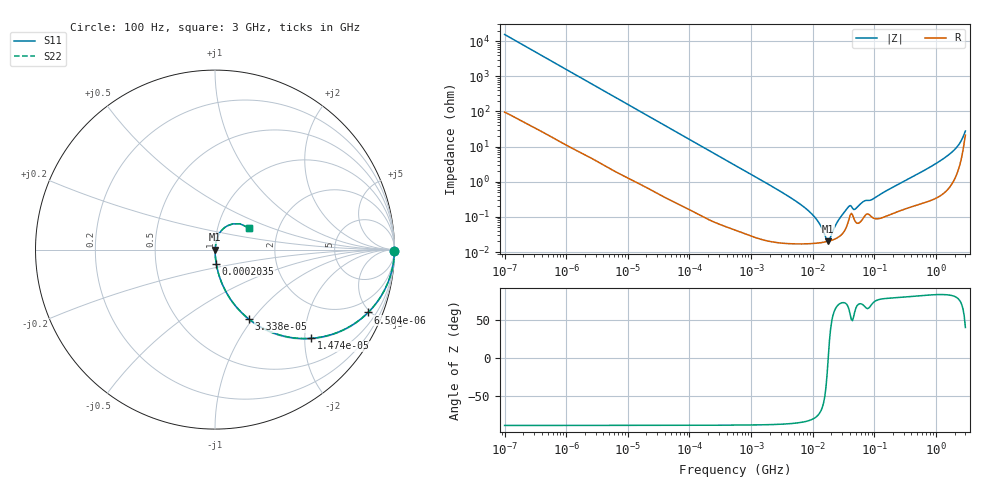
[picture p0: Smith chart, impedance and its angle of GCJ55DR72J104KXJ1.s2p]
!Murata Part Number: GCJ55DR72J104KXJ1
!These Parameters are Measured in Series Mode Connection
!Data Generated on Mar 13, 2026
!  o--ll--o
!Port1  Port2
!  o------o
!Operation Temp=25[degC], DC Bias Voltage=0[V]
!Freq. Start=100[Hz] Stop=3[GHz] 401[Steps]
# Hz S RI R 50
!Freq.(Hz) S11(Real) S11(Imag) S21(Real) S21(Imag) S12(Real) S12(Imag) S22(Real) S22(Imag)
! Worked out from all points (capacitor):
!   401 points, 100 Hz to 3 GHz, reference 50 ohm
!   read as one part in series: C = 103 nF near 109 Hz
!   lowest |Z| = 20.2 mohm at 17.89 MHz (marker M1)
!   series resonance near 17.83 MHz, so ESL is about 780 pH
!   S11 on the Smith chart (normalised r, x): 100 Hz: open; 6.504 kHz: 1.04, -4.85; 14.74 kHz: 1.02, -2.15; 33.38 kHz: 1.01, -0.95; 203.5 kHz: 1.00, -0.16; 3 GHz: 1.42, +0.36
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100  0.9999 -0.00646  8.14e-05 0.00646  8.14e-05 0.00646  0.9999 -0.00646
1788  0.9864 -0.1124  0.0136 0.1124  0.0136 0.1124  0.9864 -0.1124
6504  0.8528 -0.3504  0.1472 0.3504  0.1472 0.3504  0.8528 -0.3504
14736  0.5359 -0.4945  0.4641 0.4945  0.4641 0.4945  0.5359 -0.4945
31977  0.2006 -0.3961  0.7994 0.3961  0.7994 0.3961  0.2006 -0.3961
33383  0.1873 -0.3858  0.8127 0.3858  0.8127 0.3858  0.1873 -0.3858
69391  0.0522 -0.2178  0.9478 0.2178  0.9478 0.2178  0.0522 -0.2178
203529  0.00702 -0.0784  0.993 0.0784  0.993 0.0784  0.00702 -0.0784
547723  0.00129 -0.0295  0.9987 0.0295  0.9987 0.0295  0.00129 -0.0295
4323298  0.000185 -0.00355  0.9998 0.00355  0.9998 0.00355  0.000185 -0.00355
9794414  0.000175 -0.00117  0.9998 0.00117  0.9998 0.00117  0.000175 -0.00117
1.268047e7  0.000182 -0.000642  0.9998 0.000642  0.9998 0.000642  0.000182 -0.000642
1.789277e7  0.000202 6.4e-06  0.9998 -6.4e-06  0.9998 -6.4e-06  0.000202 6.4e-06
2.52476e7  0.000256 0.000684  0.9997 -0.000684  0.9997 -0.000684  0.000256 0.000684
3.71925e7  0.000674 0.00172  0.9993 -0.00172  0.9993 -0.00172  0.000674 0.00172
5.026954e7  0.000697 0.00159  0.9993 -0.00159  0.9993 -0.00159  0.000697 0.00159
6.794454e7  0.000996 0.00261  0.999 -0.00261  0.999 -0.00261  0.000996 0.00261
9.183415e7  0.000985 0.00296  0.999 -0.00296  0.999 -0.00296  0.000985 0.00296
1.751444e8  0.00117 0.00605  0.9988 -0.00605  0.9988 -0.00605  0.00117 0.00605
1.382454e9  0.00712 0.0471  0.9929 -0.0471  0.9929 -0.0471  0.00712 0.0471
2.126076e9  0.0224 0.0872  0.9776 -0.0872  0.9776 -0.0872  0.0224 0.0872
3e9  0.1917 0.12  0.8083 -0.12  0.8083 -0.12  0.1917 0.12
